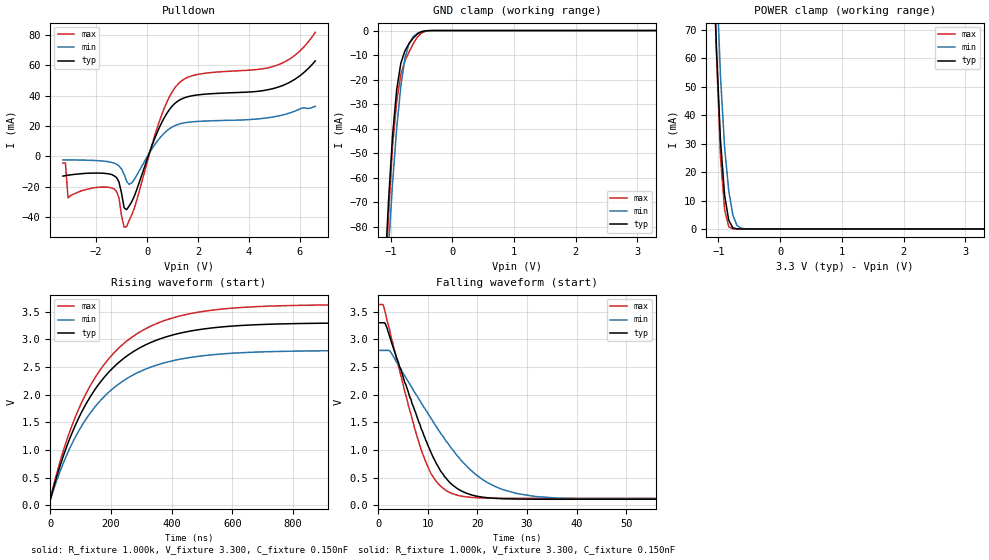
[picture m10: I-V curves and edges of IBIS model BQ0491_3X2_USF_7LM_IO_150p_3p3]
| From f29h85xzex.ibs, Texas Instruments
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|   Model BQ0491_3X2_USF_7LM_IO_150p_3p3
[Model]   BQ0491_3X2_USF_7LM_IO_150p_3p3
Model_type   I/O_open_drain
Polarity   Non-Inverting
Enable   Active-Low
Vinl =   0.800V
Vinh =   2.000V
Vmeas =  1.650V
Cref =   0.150nF
Rref =   1.000k
Vref =   3.300V
|   typ   min   max
C_comp   1.084pF   1.003pF   1.123pF
[Model Spec]
Vinh   2.000V   2.000V   2.000V
Vinl   0.800V   0.800V   0.800V
[Temperature Range]   25   155   -40
[Voltage Range]   3.300V   2.800V   3.630V
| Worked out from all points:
|   slope of the pulldown table from 0 to 0.495 V, typ, clamps not added: 22.9 ohm
|   GND clamp passes 1 mA (typ) near -0.53 V on its own axis
|   POWER clamp passes 1 mA (typ) near -0.78 V on its own axis
|   rising waveform, R_fixture 1.000k, V_fixture 3.300, C_fixture 0.150nF: 20-80 % time 209ns typ, 209ns min, 209ns max; typ from 0.109 V to 3.3 V
|   falling waveform, R_fixture 1.000k, V_fixture 3.300, C_fixture 0.150nF: 20-80 % time 8.05ns typ, 12.7ns min, 6.44ns max; typ from 3.3 V to 0.109 V
[Pulldown]
|Voltage   I(typ)   I(min)   I(max)
-3.3V     -13.02mA   -2.341mA   -4.302mA
-3.2V     -12.73mA   -2.337mA   -4.378mA
-3.1V     -12.44mA   -2.348mA   -27.4mA
-1.3V     -12.73mA   -4.396mA   -21.37mA
-1.1V     -16.92mA   -6.309mA   -27.33mA
-900mV    -33.88mA   -11.82mA   -46.69mA
-800mV    -35.17mA   -16.44mA   -46.34mA
-600mV    -29.93mA   -17.47mA   -38.61mA
500mV     19.62mA    12.09mA    23.89mA
1.2V      36.37mA    21.01mA    47.41mA
5.1V      45.45mA    26.46mA    60.14mA
6.6V      62.95mA    33.05mA    81.82mA
[GND_clamp]
|Voltage   I(typ)   I(min)   I(max)
-3.3V     -1.477A    -1.275A    -1.767A
-1.1V     -102.3mA   -117.4mA   -113.6mA
-1.033V   -69.62mA   -88.44mA   -75.69mA
-967mV    -42.73mA   -62.13mA   -47.02mA
-900mV    -23.96mA   -39.74mA   -28.87mA
-833mV    -13.32mA   -22.64mA   -17.88mA
-767mV    -8.289mA   -11.35mA   -12.33mA
-700mV    -5.352mA   -5.293mA   -8.734mA
-567mV    -1.458mA   -1.135mA   -2.736mA
-433mV    -112.7uA   -134.1uA   -294.8uA
-300mV    -3.58uA    -9.04uA    -6.616uA
3.3V      0A         0A         0A
[POWER_clamp]
|Voltage   I(typ)   I(min)   I(max)
-3.3V     1.901A     2.191A     2.069A
-1.1V     105.6mA    134.8mA    109.4mA
-1.033V   63.91mA    89.93mA    62.06mA
-967mV    31.18mA    53.67mA    25.42mA
-900mV    11.84mA    28.57mA    6.708mA
-833mV    3.029mA    13.38mA    772.2uA
-767mV    401uA      4.887mA    44.81uA
-700mV    39.92uA    1.256mA    4.586uA
-633mV    5.005uA    258uA      1.414uA
-567mV    1.06uA     50.07uA    519.2nA
3.3V      0A         0A         0A
[Ramp]
| variable   typ   min   max
dV/dt_r   1.914/1.296n   1.615/1.263n   2.103/1.336n
dV/dt_f   1.914/0.125n   1.615/0.208n   2.103/98.310p
R_load = 1.000k
[Rising Waveform]
R_fixture= 1.000k
V_fixture= 3.300
V_fixture_min= 2.800
V_fixture_max= 3.630
C_fixture= 0.150nF
|time   V(typ)   V(min)   V(max)
0s        109.4mV    108.1mV    125.7mV
36.5ns    784.1mV    672.7mV    869.8mV
73ns      1.325V     1.13V      1.462V
113.2ns   1.787V     1.52V      1.969V
156.6ns   2.165V     1.84V      2.384V
258.6ns   2.723V     2.312V     2.996V
390.6ns   3.059V     2.596V     3.366V
535.6ns   3.208V     2.722V     3.529V
747.6ns   3.277V     2.781V     3.605V
2us       3.3V       2.8V       3.63V
[Falling Waveform]
R_fixture= 1.000k
V_fixture= 3.300
V_fixture_min= 2.800
V_fixture_max= 3.630
C_fixture= 0.150nF
|time   V(typ)   V(min)   V(max)
0s        3.3V       2.8V       3.63V
1ns       3.3V       2.8V       3.622V
1.7ns     3.223V     2.8V       3.379V
7.3ns     1.728V     2.049V     1.403V
10.7ns    944.1mV    1.565V     567.4mV
15ns      367.9mV    1.011V     209.4mV
22.3ns    134.7mV    397.1mV    129.5mV
36ns      109.6mV    130.8mV    125.7mV
66.9ns    109.3mV    108.2mV    125.7mV
2us       109.3mV    108.1mV    125.7mV
